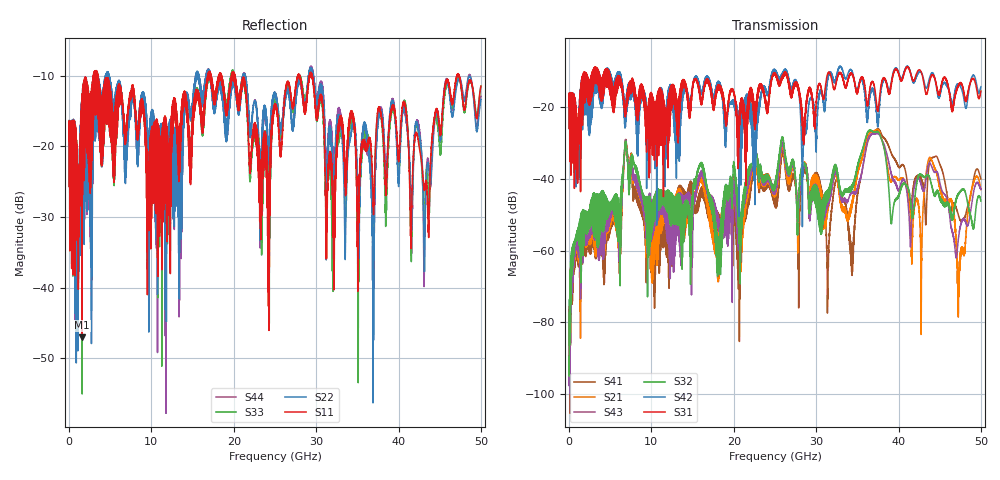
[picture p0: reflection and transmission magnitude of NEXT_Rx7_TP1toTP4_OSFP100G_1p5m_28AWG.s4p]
! Touchstone data
! Created: 27-Feb-2019 by IdEM 12 (12.1.0)
! COMMENTS
!  Created Wed Feb 27 09:43:39 2019
!  64 Port Network Data from SP1.SP block
!  freq  magS1_1  angS1_1  magS1_2  angS1_2  magS1_3  angS1_3  magS1_4  angS1_4
!  magS1_5  angS1_5  magS1_6  angS1_6  magS1_7  angS1_7  magS1_8  angS1_8
!  magS1_9  angS1_9  magS1_10  angS1_10  magS1_11  angS1_11  magS1_12  angS1_12
!  magS1_13  angS1_13  magS1_14  angS1_14  magS1_15  angS1_15  magS1_16  angS1_16
!  magS1_17  angS1_17  magS1_18  angS1_18  magS1_19  angS1_19  magS1_20  angS1_20
!  magS1_21  angS1_21  magS1_22  angS1_22  magS1_23  angS1_23  magS1_24  angS1_24
!  magS1_25  angS1_25  magS1_26  angS1_26  magS1_27  angS1_27  magS1_28  angS1_28
!  magS1_29  angS1_29  magS1_30  angS1_30  magS1_31  angS1_31  magS1_32  angS1_32
!  magS1_33  angS1_33  magS1_34  angS1_34  magS1_35  angS1_35  magS1_36  angS1_36
!  magS1_37  angS1_37  magS1_38  angS1_38  magS1_39  angS1_39  magS1_40  angS1_40
!  magS1_41  angS1_41  magS1_42  angS1_42  magS1_43  angS1_43  magS1_44  angS1_44
!  magS1_45  angS1_45  magS1_46  angS1_46  magS1_47  angS1_47  magS1_48  angS1_48
!  magS1_49  angS1_49  magS1_50  angS1_50  magS1_51  angS1_51  magS1_52  angS1_52
!  magS1_53  angS1_53  magS1_54  angS1_54  magS1_55  angS1_55  magS1_56  angS1_56
!  magS1_57  angS1_57  magS1_58  angS1_58  magS1_59  angS1_59  magS1_60  angS1_60
!  magS1_61  angS1_61  magS1_62  angS1_62  magS1_63  angS1_63  magS1_64  angS1_64
!  magS2_1  angS2_1  magS2_2  angS2_2  magS2_3  angS2_3  magS2_4  angS2_4
!  magS2_5  angS2_5  magS2_6  angS2_6  magS2_7  angS2_7  magS2_8  angS2_8
!  magS2_9  angS2_9  magS2_10  angS2_10  magS2_11  angS2_11  magS2_12  angS2_12
!  magS2_13  angS2_13  magS2_14  angS2_14  magS2_15  angS2_15  magS2_16  angS2_16
!  magS2_17  angS2_17  magS2_18  angS2_18  magS2_19  angS2_19  magS2_20  angS2_20
!  magS2_21  angS2_21  magS2_22  angS2_22  magS2_23  angS2_23  magS2_24  angS2_24
!  magS2_25  angS2_25  magS2_26  angS2_26  magS2_27  angS2_27  magS2_28  angS2_28
!  magS2_29  angS2_29  magS2_30  angS2_30  magS2_31  angS2_31  magS2_32  angS2_32
!  magS2_33  angS2_33  magS2_34  angS2_34  magS2_35  angS2_35  magS2_36  angS2_36
!  magS2_37  angS2_37  magS2_38  angS2_38  magS2_39  angS2_39  magS2_40  angS2_40
!  magS2_41  angS2_41  magS2_42  angS2_42  magS2_43  angS2_43  magS2_44  angS2_44
!  magS2_45  angS2_45  magS2_46  angS2_46  magS2_47  angS2_47  magS2_48  angS2_48
!  magS2_49  angS2_49  magS2_50  angS2_50  magS2_51  angS2_51  magS2_52  angS2_52
!  magS2_53  angS2_53  magS2_54  angS2_54  magS2_55  angS2_55  magS2_56  angS2_56
!  magS2_57  angS2_57  magS2_58  angS2_58  magS2_59  angS2_59  magS2_60  angS2_60
!  magS2_61  angS2_61  magS2_62  angS2_62  magS2_63  angS2_63  magS2_64  angS2_64
!  magS3_1  angS3_1  magS3_2  angS3_2  magS3_3  angS3_3  magS3_4  angS3_4
!  magS3_5  angS3_5  magS3_6  angS3_6  magS3_7  angS3_7  magS3_8  angS3_8
!  magS3_9  angS3_9  magS3_10  angS3_10  magS3_11  angS3_11  magS3_12  angS3_12
!  magS3_13  angS3_13  magS3_14  angS3_14  magS3_15  angS3_15  magS3_16  angS3_16
!  magS3_17  angS3_17  magS3_18  angS3_18  magS3_19  angS3_19  magS3_20  angS3_20
!  magS3_21  angS3_21  magS3_22  angS3_22  magS3_23  angS3_23  magS3_24  angS3_24
!  magS3_25  angS3_25  magS3_26  angS3_26  magS3_27  angS3_27  magS3_28  angS3_28
!  magS3_29  angS3_29  magS3_30  angS3_30  magS3_31  angS3_31  magS3_32  angS3_32
!  magS3_33  angS3_33  magS3_34  angS3_34  magS3_35  angS3_35  magS3_36  angS3_36
!  magS3_37  angS3_37  magS3_38  angS3_38  magS3_39  angS3_39  magS3_40  angS3_40
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# Hz S MA R 50
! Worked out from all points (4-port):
!   5000 points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, 10 MHz to 50 GHz, reference 50 ohm
!   strongest paths, dB at 10 MHz, 12.51 GHz, 25.01 GHz, 37.51 GHz, 50 GHz:
!     S31: -19.6, -16.2, -10.8, -21.0, -15.4
!     S42: -19.6, -16.6, -9.8, -25.4, -14.2
!     S32: -89.7, -44.2, -41.5, -26.9, -46.2
!     S43: -91.8, -47.3, -44.1, -27.3, -42.8
!     S21: -91.5, -45.2, -44.0, -26.2, -42.9
!     S41: -92.3, -47.3, -47.7, -26.0, -40.0
!   lowest |S11| = -47.1 dB at 1.59 GHz (marker M1), VSWR 1.01, Z = 49.7 + j0.298 ohm
!   |S11| at or under -10 dB: 3.482 GHz to 16.85 GHz (13.37 GHz wide, 132 % of centre); 20.15 GHz to 27.79 GHz (7.635 GHz wide, 31.9 % of centre); 29.53 GHz to 47.08 GHz (17.55 GHz wide, 45.8 % of centre)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
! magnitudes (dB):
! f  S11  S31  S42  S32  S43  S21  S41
! 10 MHz  -19.2  -19.6  -19.6  -89.7  -91.8  -91.5  -92.3
! 1.59 GHz  -47.1  -24.2  -24.4  -56.2  -55.2  -55.0  -54.3
! 25.92 GHz  -17.6  -11.8  -11.0  -28.2  -29.8  -30.2  -32.4
! 34.32 GHz  -15.8  -10.4  -9.7  -41.8  -43.9  -47.6  -62.1
! 37.39 GHz  -15.9  -19.8  -22.2  -26.7  -27.1  -26.2  -26.2
! 47.33 GHz  -9.9  -13.7  -13.5  -43.8  -55.5  -68.0  -50.5
! 50 GHz  -11.5  -15.4  -14.2  -46.2  -42.8  -42.9  -40.0
